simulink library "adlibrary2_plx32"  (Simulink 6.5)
undefined symbols (not defined in the file or in its folder): Black, blackbox2, blue, Box, clock_ratio, gcbh, Inactive, lbif32_plx_config, program, VER_STRING_GOES_HERE, white, xbsIndex_r4, xlBlockLoadCallback
libraries: xbsIndex_r4 x35, adlibrary2_plx32 x1

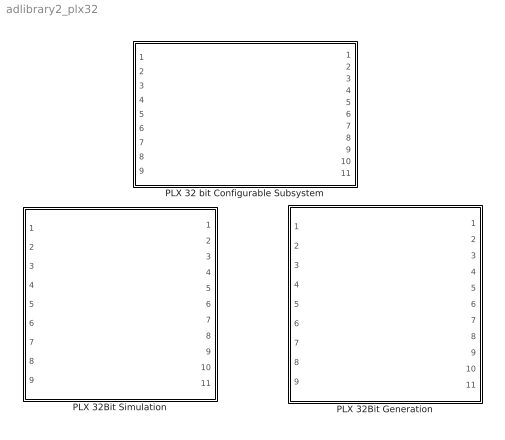
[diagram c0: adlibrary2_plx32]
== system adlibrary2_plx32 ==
  PLX 32 bit Configurable Subsystem : Subsystem  Tag=configX  BlockChoice=PLX 32Bit Simulation  mask{program=program, clock_ratio=clock_ratio}
      mask prompts: program "Local Bus Script Program"; clock_ratio "Clock Ratio"
  PLX 32Bit Generation : Subsystem
  PLX 32Bit Simulation : Subsystem  mask{program=program, clock_ratio=clock_ratio}
      mask prompts: program "Local Bus Script Program"; clock_ratio "Clock Ratio"

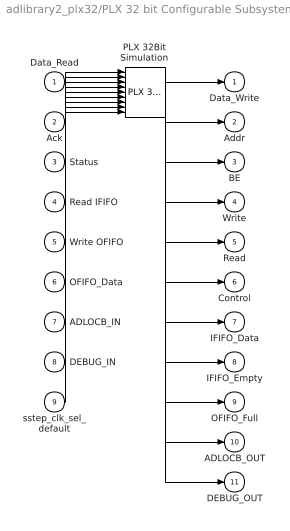
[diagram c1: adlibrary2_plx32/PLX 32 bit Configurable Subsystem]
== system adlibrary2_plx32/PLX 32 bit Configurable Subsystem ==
  Data_Read : Inport
  Ack : Inport  Port=2
  Status : Inport  Port=3
  Read IFIFO : Inport  Port=4
  Write OFIFO : Inport  Port=5
  OFIFO_Data : Inport  Port=6
  ADLOCB_IN : Inport  Port=7
  DEBUG_IN : Inport  Port=8
  sstep_clk_sel_default : Inport  Port=9
  PLX 32Bit Simulation : adlibrary2_plx32/PLX 32Bit Simulation  SystemSampleTime=-1  program=program  clock_ratio=clock_ratio
  Data_Write : Outport
  Addr : Outport  Port=2
  BE : Outport  Port=3
  Write : Outport  Port=4
  Read : Outport  Port=5
  Control : Outport  Port=6
  IFIFO_Data : Outport  Port=7
  IFIFO_Empty : Outport  Port=8
  OFIFO_Full : Outport  Port=9
  ADLOCB_OUT : Outport  Port=10
  DEBUG_OUT : Outport  Port=11
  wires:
  Data_Read/1 -> PLX 32Bit Simulation/1
  Ack/1 -> PLX 32Bit Simulation/2
  Status/1 -> PLX 32Bit Simulation/3
  Read IFIFO/1 -> PLX 32Bit Simulation/4
  Write OFIFO/1 -> PLX 32Bit Simulation/5
  OFIFO_Data/1 -> PLX 32Bit Simulation/6
  ADLOCB_IN/1 -> PLX 32Bit Simulation/7
  DEBUG_IN/1 -> PLX 32Bit Simulation/8
  sstep_clk_sel_default/1 -> PLX 32Bit Simulation/9
  PLX 32Bit Simulation/1 -> Data_Write/1
  PLX 32Bit Simulation/2 -> Addr/1
  PLX 32Bit Simulation/3 -> BE/1
  PLX 32Bit Simulation/4 -> Write/1
  PLX 32Bit Simulation/5 -> Read/1
  PLX 32Bit Simulation/6 -> Control/1
  PLX 32Bit Simulation/7 -> IFIFO_Data/1
  PLX 32Bit Simulation/8 -> IFIFO_Empty/1
  PLX 32Bit Simulation/9 -> OFIFO_Full/1
  PLX 32Bit Simulation/10 -> ADLOCB_OUT/1
  PLX 32Bit Simulation/11 -> DEBUG_OUT/1

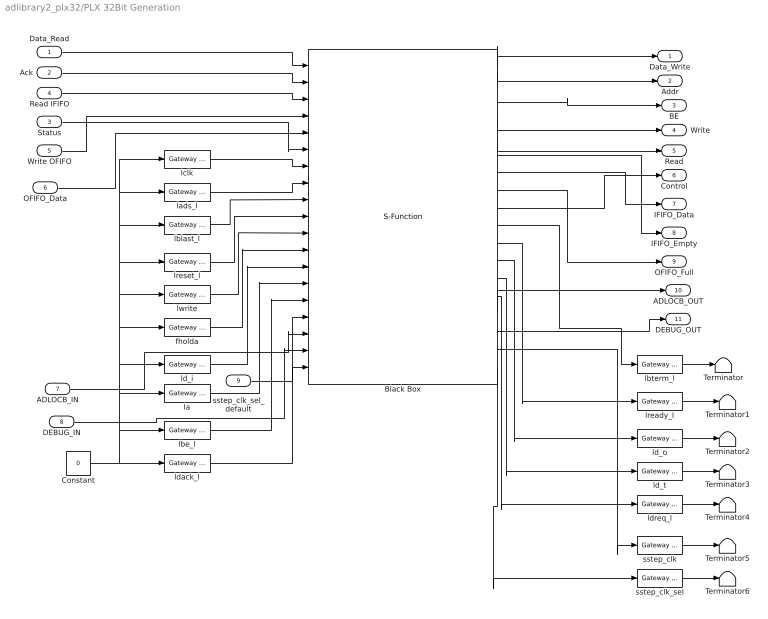
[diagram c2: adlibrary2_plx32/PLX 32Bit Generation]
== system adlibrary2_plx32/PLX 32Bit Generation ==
  Data_Read : Inport
  Ack : Inport  Port=2
  Status : Inport  Port=3
  Read IFIFO : Inport  Port=4
  Write OFIFO : Inport  Port=5
  OFIFO_Data : Inport  Port=6
  ADLOCB_IN : Inport  Port=7
  DEBUG_IN : Inport  Port=8
  sstep_clk_sel_default : Inport  Port=9
  Black Box : S-Function  AncestorBlock=xbsIndex_r4/Black Box  LoadFcn=xlBlockLoadCallback(gcbh);  FunctionName=sysgen  Parameters=ptable_  mask(Xilinx Black Box Block){infoedit=Incorporates black box HDL and simulation model into a System Generator design.<P><P>You must supply a Black Box with certain information about the HDL component you would like to bring into System Generator. This information is provided through a Matlab function.<P><P>When "Simulation mode" is set to "Inactive", you will typically want to provide a separate simulation model by using a Simulation 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, init_code=lbif32_plx_config, sim_method=Inactive, sim_method_sgadvanced=, engine_block=, xl_use_area=on, xl_use_area_sgadvanced=, xl_area=[576,805, 3, 586, 0, 0, 162], block_version=VER_STRING_GOES_HERE, has_advanced_control=0, sggui_pos=20,20,356,367, block_type=blackbox2, sg_icon_stat=230,408,19,18,white,blue,0,24d5618f, sg_mask_display=fprintf('','COMMENT: begin icon graphics '); patch([0 230 230 0 ],[0 0 408 408 ],[0.77 0.82 0.91]); patch([54 16 70 16 54 115 131 147 212 161 112 76 130 76 112 161 212 147 131 115 54 ],[114 152 206 260 298 298 282 298 298 247 296 260 206 152 116 165 114 114 130 114 114 ],[0.98 0.96 0.92]); plot([0 0 230 230 0 ],[0 408 408 0 0 ]); fprintf('','COMMENT: end icon graphics');  fprintf('','COMMENT: begi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, sg_list_contents=}
      mask prompts: infoedit ""; init_code "Block configuration m-function"; sim_method "Simulation mode"; engine_block "HDL co-simulator to use  (specify helper block by name)"; xl_use_area "Define FPGA area for resource estimation"; xl_area "FPGA area [slices, FFs, BRAMs, LUTs, IOBs, emb. mults, TBUFs]"; block_version ""; has_advanced_control ""; sggui_pos ""; block_type ""; sg_icon_stat ""; sg_mask_display ""; sg_list_contents ""
      mask help: Incorporates black box HDL and simulation model into a System Generator design. You must supply a Black Box with certain information about the HDL component you would like to bring into System Generator. This information is provided through a Matlab function. When "Simulation mode" is set to "Inactive", you will typically want to provide a separate simulation model by using a Simulation Multiplexer. When "Simulation mode" is set to "External co-simulator", you must include a ModelSim block in the design.
      mask init:
      | xlMungeMaskParams;
      | 
      | mdlPath = xlGetMdlDir(bdroot);
      | 
      | refBlk = get_param(gcb,'referenceBlock');
      | if (isempty(refBlk) | strncmp(refBlk,'xbsIndex',8))
      | srcPath = mdlPath;
      | else
      | srcPath = xlPathToReference;
      | if (isempty(srcPath))
      | srcPath = mdlPath;
      | end
      | end
      | 
      | if (sim_method==3)
      | validEngineBlock = 0;
      | try
      | engineBlock = xlBlockNameRelPath(get_param(gcb,'Parent'),engine_block);
      | catch
      | engineBlock = '//';
      | end
      | try 
      | engineWorkDir = get_param(engineBlock,'dir');
      | validEngineBlock = 1;
      | engine_handle = get_param(engineBlock,'Handle');
      | catch
      | end
      | end
      | 
      | % build black box config function
      | block_config = ['sysgen:black_box_config:' init_code];
      | 
      | serialized_declarations = '{''engine_handle''=>''Double'',''sim_method''=>''Int'',''validEngineBlock''=>''Int'',''engineWorkDir''=>''String'',''engine_block''=>''String'',''init_code''=>''String'',''mdlPath''=>''String'',''srcPath''=>''String'',''block_config''=>''String'',}';
      | ptable_ = xlblockprep(get_param(gcb, 'MaskWSVariables'));
  Constant : Constant  Value=0  OutDataType=sfix(16)  ConRadixGroup=Use specified scaling  OutScaling=2^0  SampleTime=inf  FramePeriod=inf
  Terminator{,1..6} (7 alike) : Terminator
  fholda : xbsIndex_r4/Gateway In  arith_type=Boolean  n_bits=8  bin_pt=6  quantization="Round  (unbiased: +/- Inf)"  overflow=Saturate  period=ad_get_simulink_period  dbl_ovrd=off  timing_constraint=None  locs_specified=off  LOCs={}  block_type=gatewayin
  la : xbsIndex_r4/Gateway In  arith_type=Unsigned  n_bits=24  bin_pt=0  quantization="Round  (unbiased: +/- Inf)"  overflow=Saturate  period=ad_get_simulink_period  dbl_ovrd=off  timing_constraint=None  locs_specified=off  LOCs={}  block_type=gatewayin
  lads_l : xbsIndex_r4/Gateway In  arith_type=Boolean  n_bits=8  bin_pt=6  quantization="Round  (unbiased: +/- Inf)"  overflow=Saturate  period=ad_get_simulink_period  dbl_ovrd=off  timing_constraint=None  locs_specified=off  LOCs={}  block_type=gatewayin
  lbe_l : xbsIndex_r4/Gateway In  arith_type=Unsigned  n_bits=4  bin_pt=0  quantization="Round  (unbiased: +/- Inf)"  overflow=Saturate  period=ad_get_simulink_period  dbl_ovrd=off  timing_constraint=None  locs_specified=off  LOCs={}  block_type=gatewayin
  lblast_l : xbsIndex_r4/Gateway In  arith_type=Boolean  n_bits=8  bin_pt=6  quantization="Round  (unbiased: +/- Inf)"  overflow=Saturate  period=ad_get_simulink_period  dbl_ovrd=off  timing_constraint=None  locs_specified=off  LOCs={}  block_type=gatewayin
  lbterm_l : xbsIndex_r4/Gateway Out  hdl_port=on  timing_constraint=None  locs_specified=off  LOCs={}  block_type=gatewayout
  lclk : xbsIndex_r4/Gateway In  arith_type=Boolean  n_bits=8  bin_pt=6  quantization="Round  (unbiased: +/- Inf)"  overflow=Saturate  period=ad_get_simulink_period  dbl_ovrd=off  timing_constraint=None  locs_specified=off  LOCs={}  block_type=gatewayin
  ld_i : xbsIndex_r4/Gateway In  arith_type=Unsigned  n_bits=32  bin_pt=0  quantization="Round  (unbiased: +/- Inf)"  overflow=Saturate  period=ad_get_simulink_period  dbl_ovrd=off  timing_constraint=None  locs_specified=off  LOCs={}  block_type=gatewayin
  ld_o : xbsIndex_r4/Gateway Out  hdl_port=on  timing_constraint=None  locs_specified=off  LOCs={}  block_type=gatewayout
  ld_t : xbsIndex_r4/Gateway Out  hdl_port=on  timing_constraint=None  locs_specified=off  LOCs={}  block_type=gatewayout
  ldack_l : xbsIndex_r4/Gateway In  arith_type=Unsigned  n_bits=2  bin_pt=0  quantization="Round  (unbiased: +/- Inf)"  overflow=Saturate  period=ad_get_simulink_period  dbl_ovrd=off  timing_constraint=None  locs_specified=off  LOCs={}  block_type=gatewayin
  ldreq_l : xbsIndex_r4/Gateway Out  hdl_port=on  timing_constraint=None  locs_specified=off  LOCs={}  block_type=gatewayout
  lready_l : xbsIndex_r4/Gateway Out  hdl_port=on  timing_constraint=None  locs_specified=off  LOCs={}  block_type=gatewayout
  lreset_l : xbsIndex_r4/Gateway In  arith_type=Boolean  n_bits=8  bin_pt=6  quantization="Round  (unbiased: +/- Inf)"  overflow=Saturate  period=ad_get_simulink_period  dbl_ovrd=off  timing_constraint=None  locs_specified=off  LOCs={}  block_type=gatewayin
  lwrite : xbsIndex_r4/Gateway In  arith_type=Boolean  n_bits=8  bin_pt=6  quantization="Round  (unbiased: +/- Inf)"  overflow=Saturate  period=ad_get_simulink_period  dbl_ovrd=off  timing_constraint=None  locs_specified=off  LOCs={}  block_type=gatewayin
  sstep_clk : xbsIndex_r4/Gateway Out  hdl_port=on  timing_constraint=None  locs_specified=off  LOCs={}  block_type=gatewayout
  sstep_clk_sel : xbsIndex_r4/Gateway Out  hdl_port=on  timing_constraint=None  locs_specified=off  LOCs={}  block_type=gatewayout
  Data_Write : Outport
  Addr : Outport  Port=2
  BE : Outport  Port=3
  Write : Outport  Port=4
  Read : Outport  Port=5
  Control : Outport  Port=6
  IFIFO_Data : Outport  Port=7
  IFIFO_Empty : Outport  Port=8
  OFIFO_Full : Outport  Port=9
  ADLOCB_OUT : Outport  Port=10
  DEBUG_OUT : Outport  Port=11
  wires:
  Data_Read/1 -> Black Box/1
  Write OFIFO/1 -> Black Box/4
  OFIFO_Data/1 -> Black Box/5
  lclk/1 -> Black Box/7
  lblast_l/1 -> Black Box/9
  lreset_l/1 -> Black Box/10
  lwrite/1 -> Black Box/11
  fholda/1 -> Black Box/12
  ld_i/1 -> Black Box/13
  la/1 -> Black Box/14
  lbe_l/1 -> Black Box/15
  ldack_l/1 -> Black Box/16
  Constant/1 -> ldack_l/1, lclk/1, lads_l/1, lblast_l/1, lreset_l/1, lwrite/1, fholda/1, ld_i/1, la/1, lbe_l/1
  lbterm_l/1 -> Terminator/1
  lready_l/1 -> Terminator1/1
  ld_o/1 -> Terminator2/1
  ld_t/1 -> Terminator3/1
  ldreq_l/1 -> Terminator4/1
  Black Box/1 -> Data_Write/1
  Black Box/2 -> Addr/1
  Black Box/3 -> BE/1
  Black Box/4 -> Write/1
  Black Box/5 -> Read/1
  Black Box/7 -> IFIFO_Data/1
  Black Box/8 -> OFIFO_Full/1
  Black Box/6 -> IFIFO_Empty/1
  Black Box/9 -> Control/1
  Black Box/10 -> lbterm_l/1
  Black Box/11 -> lready_l/1
  Black Box/12 -> ld_o/1
  Black Box/13 -> ld_t/1
  Black Box/14 -> ldreq_l/1
  Ack/1 -> Black Box/2
  Read IFIFO/1 -> Black Box/3
  lads_l/1 -> Black Box/8
  Status/1 -> Black Box/6
  ADLOCB_IN/1 -> Black Box/17
  Black Box/15 -> ADLOCB_OUT/1
  sstep_clk/1 -> Terminator5/1
  sstep_clk_sel/1 -> Terminator6/1
  Black Box/17 -> sstep_clk/1
  Black Box/18 -> sstep_clk_sel/1
  Black Box/16 -> DEBUG_OUT/1
  DEBUG_IN/1 -> Black Box/18
  sstep_clk_sel_default/1 -> Black Box/19

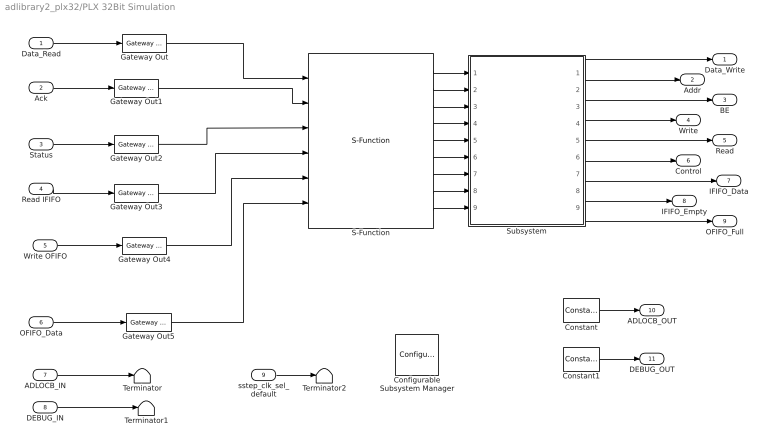
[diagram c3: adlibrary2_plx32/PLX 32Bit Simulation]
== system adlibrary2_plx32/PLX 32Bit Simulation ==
  Data_Read : Inport
  Ack : Inport  Port=2
  Status : Inport  Port=3
  Read IFIFO : Inport  Port=4
  Write OFIFO : Inport  Port=5
  OFIFO_Data : Inport  Port=6
  ADLOCB_IN : Inport  Port=7
  DEBUG_IN : Inport  Port=8
  sstep_clk_sel_default : Inport  Port=9
  Configurable Subsystem Manager : xbsIndex_r4/Configurable Subsystem Manager  Tag=xcfgMgr  block_type=configsubsys
  Constant : xbsIndex_r4/Constant  arith_type=Unsigned  const=0  n_bits=34  bin_pt=0  explicit_period=on  period=ad_get_simulink_period  equ=P=C  opselect=C  inp2=PCIN>>17  opr=+  inp1=P  carry=CIN  dbl_ovrd=off  block_type=constant
  Constant1 : xbsIndex_r4/Constant  arith_type=Unsigned  const=0  n_bits=40  bin_pt=0  explicit_period=on  period=ad_get_simulink_period  equ=P=C  opselect=C  inp2=PCIN>>17  opr=+  inp1=P  carry=CIN  dbl_ovrd=off  block_type=constant
  Gateway Out{,1..5} (6 alike) : xbsIndex_r4/Gateway Out  hdl_port=off  timing_constraint=None  locs_specified=off  LOCs={}  block_type=gatewayout
  S-Function : S-Function  FunctionName=lbif_plx32  Parameters=program,clock_ratio
  Subsystem : Subsystem
  Terminator : Terminator
  Terminator1 : Terminator
  Terminator2 : Terminator
  Data_Write : Outport
  Addr : Outport  Port=2
  BE : Outport  Port=3
  Write : Outport  Port=4
  Read : Outport  Port=5
  Control : Outport  Port=6
  IFIFO_Data : Outport  Port=7
  IFIFO_Empty : Outport  Port=8
  OFIFO_Full : Outport  Port=9
  ADLOCB_OUT : Outport  Port=10
  DEBUG_OUT : Outport  Port=11
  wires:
  Subsystem/2(Out2) -> Addr/1
  Subsystem/1(Out1) -> Data_Write/1
  S-Function/2 -> Subsystem/2(In2)
  S-Function/1 -> Subsystem/1(In1)
  Gateway Out5/1 -> S-Function/6
  Gateway Out4/1 -> S-Function/5
  Gateway Out3/1 -> S-Function/4
  Gateway Out2/1 -> S-Function/3
  Gateway Out1/1 -> S-Function/2
  Gateway Out/1 -> S-Function/1
  OFIFO_Data/1 -> Gateway Out5/1
  Write OFIFO/1 -> Gateway Out4/1
  Read IFIFO/1 -> Gateway Out3/1
  Status/1 -> Gateway Out2/1
  Ack/1 -> Gateway Out1/1
  Data_Read/1 -> Gateway Out/1
  S-Function/3 -> Subsystem/3(In9)
  Subsystem/3(Out9) -> BE/1
  S-Function/4 -> Subsystem/4(In3)
  S-Function/5 -> Subsystem/5(In4)
  S-Function/6 -> Subsystem/6(In5)
  S-Function/7 -> Subsystem/7(In6)
  S-Function/8 -> Subsystem/8(In7)
  S-Function/9 -> Subsystem/9(In8)
  Subsystem/4(Out3) -> Write/1
  Subsystem/5(Out4) -> Read/1
  Subsystem/6(Out5) -> Control/1
  Subsystem/7(Out6) -> IFIFO_Data/1
  Subsystem/8(Out7) -> IFIFO_Empty/1
  Subsystem/9(Out8) -> OFIFO_Full/1
  ADLOCB_IN/1 -> Terminator/1
  Constant/1 -> ADLOCB_OUT/1
  DEBUG_IN/1 -> Terminator1/1
  Constant1/1 -> DEBUG_OUT/1
  sstep_clk_sel_default/1 -> Terminator2/1

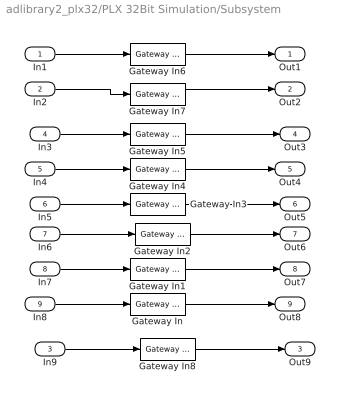
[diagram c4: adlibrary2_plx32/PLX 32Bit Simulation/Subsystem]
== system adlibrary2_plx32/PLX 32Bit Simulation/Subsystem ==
  In1 : Inport
  In2 : Inport  Port=2
  In9 : Inport  Port=3
  In3 : Inport  Port=4
  In4 : Inport  Port=5
  In5 : Inport  Port=6
  In6 : Inport  Port=7
  In7 : Inport  Port=8
  In8 : Inport  Port=9
  Gateway In{,1,4..5} (4 alike) : xbsIndex_r4/Gateway In  arith_type=Boolean  n_bits=8  bin_pt=6  quantization="Round  (unbiased: +/- Inf)"  overflow=Saturate  period=ad_get_simulink_period  dbl_ovrd=off  timing_constraint=None  locs_specified=off  LOCs={}  block_type=gatewayin
  Gateway In2 : xbsIndex_r4/Gateway In  arith_type=Unsigned  n_bits=32  bin_pt=0  quantization="Round  (unbiased: +/- Inf)"  overflow=Saturate  period=ad_get_simulink_period  dbl_ovrd=off  timing_constraint=None  locs_specified=off  LOCs={}  block_type=gatewayin
  Gateway In3 : xbsIndex_r4/Gateway In  arith_type=Unsigned  n_bits=32  bin_pt=0  quantization="Round  (unbiased: +/- Inf)"  overflow=Saturate  period=ad_get_simulink_period  dbl_ovrd=off  timing_constraint=None  locs_specified=off  LOCs={}  block_type=gatewayin
  Gateway In6 : xbsIndex_r4/Gateway In  arith_type=Unsigned  n_bits=32  bin_pt=0  quantization="Round  (unbiased: +/- Inf)"  overflow=Saturate  period=ad_get_simulink_period  dbl_ovrd=off  timing_constraint=None  locs_specified=off  LOCs={}  block_type=gatewayin
  Gateway In7 : xbsIndex_r4/Gateway In  arith_type=Unsigned  n_bits=16  bin_pt=0  quantization="Round  (unbiased: +/- Inf)"  overflow=Saturate  period=ad_get_simulink_period  dbl_ovrd=off  timing_constraint=None  locs_specified=off  LOCs={}  block_type=gatewayin
  Gateway In8 : xbsIndex_r4/Gateway In  arith_type=Unsigned  n_bits=4  bin_pt=0  quantization="Round  (unbiased: +/- Inf)"  overflow=Saturate  period=ad_get_simulink_period  dbl_ovrd=off  timing_constraint=None  locs_specified=off  LOCs={}  block_type=gatewayin
  Out1 : Outport
  Out2 : Outport  Port=2
  Out9 : Outport  Port=3
  Out3 : Outport  Port=4
  Out4 : Outport  Port=5
  Out5 : Outport  Port=6
  Out6 : Outport  Port=7
  Out7 : Outport  Port=8
  Out8 : Outport  Port=9
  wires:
  Gateway In8/1 -> Out9/1
  In9/1 -> Gateway In8/1
  Gateway In6/1 -> Out1/1
  Gateway In7/1 -> Out2/1
  Gateway In5/1 -> Out3/1
  Gateway In4/1 -> Out4/1
  Gateway In3/1 -> Out5/1
  Gateway In2/1 -> Out6/1
  Gateway In1/1 -> Out7/1
  Gateway In/1 -> Out8/1
  In8/1 -> Gateway In/1
  In7/1 -> Gateway In1/1
  In6/1 -> Gateway In2/1
  In5/1 -> Gateway In3/1
  In4/1 -> Gateway In4/1
  In3/1 -> Gateway In5/1
  In2/1 -> Gateway In7/1
  In1/1 -> Gateway In6/1
